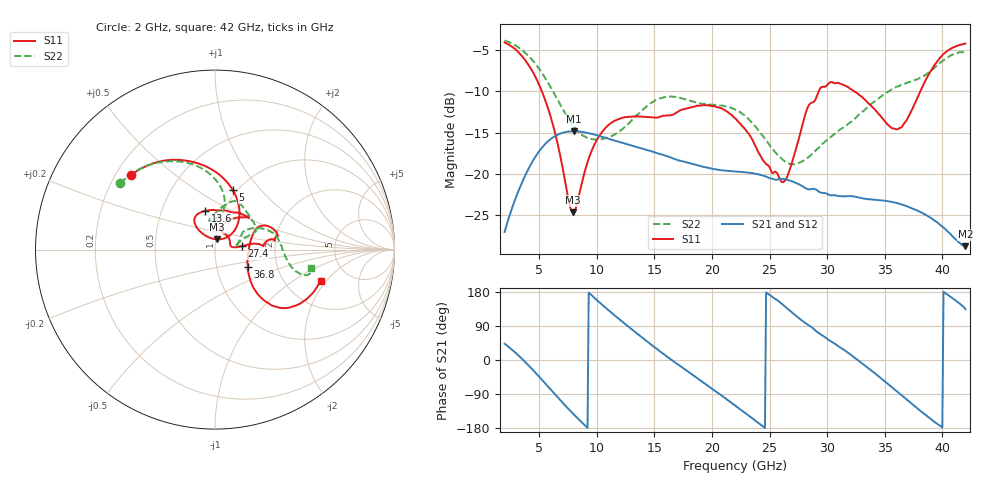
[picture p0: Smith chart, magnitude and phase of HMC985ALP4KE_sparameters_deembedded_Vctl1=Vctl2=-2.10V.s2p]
!s2p File: Measurements: S11, S21, S12, S22
# GHz S dB R 50.0
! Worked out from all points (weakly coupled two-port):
!   401 points, 2 GHz to 42 GHz, reference 50 ohm
!   highest |S21| = -14.83 dB at 8 GHz (marker M1); lowest = -28.8 dB at 42 GHz (marker M2)
!   lowest |S11| = -24.7 dB at 7.9 GHz (marker M3), VSWR 1.12, Z = 50.6 + j5.85 ohm
!   |S11| at or under -10 dB: 5.239 GHz to 29.26 GHz (24.03 GHz wide, 139 % of centre); 32.35 GHz to 38.08 GHz (5.735 GHz wide, 16.3 % of centre)
!   |S22| runs from -18.9 to -3.8 dB; largest |S21 - S12| = 0.00019
!   S11 on the Smith chart (normalised r, x): 2 GHz: 0.26, +0.36; 5 GHz: 0.95, +0.72; 13.6 GHz: 0.82, +0.37; 27.4 GHz: 1.35, +0.05; 36.8 GHz: 1.41, -0.29; 42 GHz: 3.16, -1.77
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2  -4.06 138.5  -27.05 43.0  -27.05 43.0  -3.82 144.9
3.5  -5.71 107.4  -21.09 3.3  -21.09 3.3  -4.98 119.5
5  -9.20 73.5  -17.25 -44.2  -17.25 -44.2  -7.26 95.5
6.6  -16.32 44.5  -15.25 -98.3  -15.26 -98.4  -11.02 79.0
7.9  -24.68 81.2  -14.84 -140.4  -14.84 -140.4  -14.08 81.1
8  -24.67 89.0  -14.83 -143.5  -14.83 -143.5  -14.26 81.9
8.7  -21.15 122.3  -14.90 -164.7  -14.91 -164.7  -15.26 88.7
10.6  -14.68 127.6  -15.55 142.3  -15.56 142.3  -15.74 101.4
13.6  -13.04 103.9  -16.79 67.4  -16.80 67.4  -12.73 82.7
15.4  -13.12 80.9  -17.56 25.0  -17.56 25.0  -10.89 70.4
19  -11.73 44.3  -19.06 -53.8  -19.06 -53.8  -11.46 44.1
22  -13.23 54.7  -19.70 -119.8  -19.70 -119.8  -12.19 23.8
24.5  -18.46 76.4  -20.24 -177.0  -20.24 -177.0  -15.55 20.4
26.1  -21.01 17.3  -20.60 147.1  -20.61 147.1  -18.22 12.0
27.4  -16.51 7.3  -21.16 114.0  -21.16 114.0  -18.79 8.3
28.7  -11.35 4.1  -21.83 85.4  -21.83 85.4  -17.55 15.1
31.1  -9.04 16.7  -22.70 34.0  -22.70 34.0  -14.67 32.1
33.3  -11.04 27.5  -23.03 -15.0  -23.03 -15.0  -12.20 28.8
35.4  -14.19 7.8  -23.34 -66.2  -23.35 -66.1  -9.96 19.3
36.8  -13.69 -28.3  -23.87 -101.6  -23.88 -101.6  -9.02 10.5
39.7  -6.08 -41.0  -26.04 -171.6  -26.05 -171.7  -6.68 -15.0
42  -4.19 -16.3  -28.77 134.2  -28.79 134.2  -5.25 -10.7
